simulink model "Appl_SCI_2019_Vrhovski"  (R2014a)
settings: Solver=ode45  StartTime=0.0  StopTime=1000  MaxStep=0.01  RelTol=1e-3
undefined symbols (not defined in the file): deg, H, kg, m, M, mm, N, rad, s, X, Y, Z
libraries: sm_lib x389, nesl_utility x69, simulink x7
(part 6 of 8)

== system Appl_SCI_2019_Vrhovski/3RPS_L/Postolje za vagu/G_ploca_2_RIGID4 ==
  ReferenceFrame : sm_lib/Frames and Transforms/Reference Frame  BlockFunction=simmechanics.library.frames_transforms.reference_frame
  Solid : sm_lib/Body Elements/Solid  InertiaType=Custom  Mass=5  MassUnits=kg  CenterOfMass=[-1.0925911726464245e-05 0 -4.4436244658035022]  CenterOfMassUnits=mm  MomentsOfInertia=[45540 79860 45540]  MomentsOfInertiaUnits=kg*mm^2  ProductsOfInertia=[0 -0.00010369999054466602 0]  ProductsOfInertiaUnits=kg*mm^2  DensityBased=on  Density=1000  DensityUnits=kg/(m^3)  GraphicType=FromGeometry  MarkerShape=Sphere  MarkerSize=10  MarkerSizeUnits=m  GraphicVisPropType=SimpleVisualProperties  GraphicDiffuseColor=[0.8 0.8 0.8]  GraphicSpecularColor=[0.5 0.5 0.5 1.0]  GraphicAmbientColor=[0.15 0.15 0.15 1.0]  GraphicEmissiveColor=[0.0 0.0 0.0 1.0]  GraphicShininess=75  GraphicOpacity=1  GeometryShape=Brick  RectangleSize=[1 1]  RectangleSizeUnits=m  BrickDimensions=[100 65 40]  BrickDimensionUnits=mm  CylinderRadius=120  CylinderRadiusUnits=mm  CylinderLength=20  CylinderLengthUnits=mm  SphereRadius=1  SphereRadiusUnits=m  EllipsoidRadii=[1 1 1]  EllipsoidRadiiUnits=m  ExtrusionCrossSection=[1 1; -1 1; -1 -1; 1 -1]  ExtrusionCrossSectionUnits=m  ExtrusionLength=1  ExtrusionLengthUnits=m  PolygonNumSides=3  PolygonOuterRadius=1  PolygonOuterRadiusUnits=m  ExtGeomFileType=STL  ExtGeomFileName=G_ploca_Default_sldprt.STL  ExtGeomFileUnits=mm  RevolutionCrossSection=[1 1; 1 -1; 2 -1; 2 1]  RevolutionCrossSectionUnits=m  RevolutionExtent=Full  RevolutionAngle=180  RevolutionAngleUnits=deg  BlockFunction=simmechanics.library.body_elements.solid
  Transform1 : sm_lib/Frames and Transforms/Rigid Transform  TranslationMethod=None  TranslationLengthUnit=mm  TranslationStandardAxis=-Z  TranslationStandardOffset=35.5  TranslationCartesianOffset="[-50.0000   86.6025         -10]"  TranslationROffset=0  TranslationROffsetUnits=m  TranslationZOffset=0  TranslationZOffsetUnits=m  TranslationThetaOffset=0  TranslationThetaOffsetUnits=deg  RotationMethod=ArbitraryAxis  RotationAngleUnits=rad  RotationStandardAxis=+Z  RotationAngle=0  RotationArbitraryAxis=[0 0 0]  FollAlignAxisA=+X  BaseAlignAxisA=+Y  FollAlignAxisB=+Y  BaseAlignAxisB=+Z  BlockFunction=simmechanics.library.frames_transforms.rigid_transform
  Transform3 : sm_lib/Frames and Transforms/Rigid Transform  TranslationMethod=None  TranslationLengthUnit=mm  TranslationStandardAxis=+Z  TranslationStandardOffset=35.5  TranslationCartesianOffset=[80.000000000002558 4.2632564145606011e-14 -32.999999999999048]  TranslationROffset=0  TranslationROffsetUnits=m  TranslationZOffset=0  TranslationZOffsetUnits=m  TranslationThetaOffset=0  TranslationThetaOffsetUnits=deg  RotationMethod=None  RotationAngleUnits=rad  RotationStandardAxis=+Z  RotationAngle=0  RotationArbitraryAxis=[0 0 0]  FollAlignAxisA=+X  BaseAlignAxisA=+Y  FollAlignAxisB=+Y  BaseAlignAxisB=+Z  BlockFunction=simmechanics.library.frames_transforms.rigid_transform
  B : PMIOPort  Port=1  Side=Left
  F : PMIOPort  Port=2  Side=Right
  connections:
  Transform3/RConn1 -- F/RConn1
  Transform3/LConn1 -- Solid/RConn1 -- ReferenceFrame/RConn1 -- Transform1/LConn1
  Transform1/RConn1 -- B/RConn1

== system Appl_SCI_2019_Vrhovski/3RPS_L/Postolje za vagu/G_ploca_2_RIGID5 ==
  ReferenceFrame : sm_lib/Frames and Transforms/Reference Frame  BlockFunction=simmechanics.library.frames_transforms.reference_frame
  Solid : sm_lib/Body Elements/Solid  InertiaType=Custom  Mass=5  MassUnits=kg  CenterOfMass=[-1.0925911726464245e-05 0 -4.4436244658035022]  CenterOfMassUnits=mm  MomentsOfInertia=[45540 79860 45540]  MomentsOfInertiaUnits=kg*mm^2  ProductsOfInertia=[0 -0.00010369999054466602 0]  ProductsOfInertiaUnits=kg*mm^2  DensityBased=on  Density=1000  DensityUnits=kg/(m^3)  GraphicType=FromGeometry  MarkerShape=Sphere  MarkerSize=10  MarkerSizeUnits=m  GraphicVisPropType=SimpleVisualProperties  GraphicDiffuseColor=[0.8 0.8 0.8]  GraphicSpecularColor=[0.5 0.5 0.5 1.0]  GraphicAmbientColor=[0.15 0.15 0.15 1.0]  GraphicEmissiveColor=[0.0 0.0 0.0 1.0]  GraphicShininess=75  GraphicOpacity=1  GeometryShape=Brick  RectangleSize=[1 1]  RectangleSizeUnits=m  BrickDimensions=[100 65 40]  BrickDimensionUnits=mm  CylinderRadius=120  CylinderRadiusUnits=mm  CylinderLength=20  CylinderLengthUnits=mm  SphereRadius=1  SphereRadiusUnits=m  EllipsoidRadii=[1 1 1]  EllipsoidRadiiUnits=m  ExtrusionCrossSection=[1 1; -1 1; -1 -1; 1 -1]  ExtrusionCrossSectionUnits=m  ExtrusionLength=1  ExtrusionLengthUnits=m  PolygonNumSides=3  PolygonOuterRadius=1  PolygonOuterRadiusUnits=m  ExtGeomFileType=STL  ExtGeomFileName=G_ploca_Default_sldprt.STL  ExtGeomFileUnits=mm  RevolutionCrossSection=[1 1; 1 -1; 2 -1; 2 1]  RevolutionCrossSectionUnits=m  RevolutionExtent=Full  RevolutionAngle=180  RevolutionAngleUnits=deg  BlockFunction=simmechanics.library.body_elements.solid
  Transform1 : sm_lib/Frames and Transforms/Rigid Transform  TranslationMethod=None  TranslationLengthUnit=mm  TranslationStandardAxis=-Z  TranslationStandardOffset=35.5  TranslationCartesianOffset="[-50.0000   86.6025         -10]"  TranslationROffset=0  TranslationROffsetUnits=m  TranslationZOffset=0  TranslationZOffsetUnits=m  TranslationThetaOffset=0  TranslationThetaOffsetUnits=deg  RotationMethod=ArbitraryAxis  RotationAngleUnits=rad  RotationStandardAxis=+Z  RotationAngle=0  RotationArbitraryAxis=[0 0 0]  FollAlignAxisA=+X  BaseAlignAxisA=+Y  FollAlignAxisB=+Y  BaseAlignAxisB=+Z  BlockFunction=simmechanics.library.frames_transforms.rigid_transform
  Transform3 : sm_lib/Frames and Transforms/Rigid Transform  TranslationMethod=None  TranslationLengthUnit=mm  TranslationStandardAxis=+Z  TranslationStandardOffset=35.5  TranslationCartesianOffset=[80.000000000002558 4.2632564145606011e-14 -32.999999999999048]  TranslationROffset=0  TranslationROffsetUnits=m  TranslationZOffset=0  TranslationZOffsetUnits=m  TranslationThetaOffset=0  TranslationThetaOffsetUnits=deg  RotationMethod=None  RotationAngleUnits=rad  RotationStandardAxis=+Z  RotationAngle=0  RotationArbitraryAxis=[0 0 0]  FollAlignAxisA=+X  BaseAlignAxisA=+Y  FollAlignAxisB=+Y  BaseAlignAxisB=+Z  BlockFunction=simmechanics.library.frames_transforms.rigid_transform
  B : PMIOPort  Port=1  Side=Left
  F : PMIOPort  Port=2  Side=Right
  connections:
  Transform1/RConn1 -- B/RConn1
  Transform1/LConn1 -- ReferenceFrame/RConn1 -- Solid/RConn1 -- Transform3/LConn1
  Transform3/RConn1 -- F/RConn1

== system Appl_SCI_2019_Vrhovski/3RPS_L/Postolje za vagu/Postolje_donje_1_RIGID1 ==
  ReferenceFrame : sm_lib/Frames and Transforms/Reference Frame  BlockFunction=simmechanics.library.frames_transforms.reference_frame
  Transform1 : sm_lib/Frames and Transforms/Rigid Transform  TranslationMethod=Cartesian  TranslationLengthUnit=mm  TranslationStandardAxis=+Z  TranslationStandardOffset=0  TranslationCartesianOffset=[-87.5 72.7 20]  TranslationROffset=0  TranslationROffsetUnits=m  TranslationZOffset=0  TranslationZOffsetUnits=m  TranslationThetaOffset=0  TranslationThetaOffsetUnits=deg  RotationMethod=None  RotationAngleUnits=rad  RotationStandardAxis=+Z  RotationAngle=2.0943951023931975  RotationArbitraryAxis=[0.57735026918962651 -0.57735026918962651 0.5773502691896244]  FollAlignAxisA=+X  BaseAlignAxisA=+Y  FollAlignAxisB=+Y  BaseAlignAxisB=+Z  BlockFunction=simmechanics.library.frames_transforms.rigid_transform
  Transform2 : sm_lib/Frames and Transforms/Rigid Transform  TranslationMethod=Cartesian  TranslationLengthUnit=mm  TranslationStandardAxis=+Z  TranslationStandardOffset=0  TranslationCartesianOffset=[87.5 72.7 20]  TranslationROffset=0  TranslationROffsetUnits=m  TranslationZOffset=0  TranslationZOffsetUnits=m  TranslationThetaOffset=0  TranslationThetaOffsetUnits=deg  RotationMethod=None  RotationAngleUnits=rad  RotationStandardAxis=+Z  RotationAngle=2.0943951023931975  RotationArbitraryAxis=[0.57735026918962651 -0.57735026918962651 0.5773502691896244]  FollAlignAxisA=+X  BaseAlignAxisA=+Y  FollAlignAxisB=+Y  BaseAlignAxisB=+Z  BlockFunction=simmechanics.library.frames_transforms.rigid_transform
  Transform3 : sm_lib/Frames and Transforms/Rigid Transform  TranslationMethod=Cartesian  TranslationLengthUnit=mm  TranslationStandardAxis=+Z  TranslationStandardOffset=0  TranslationCartesianOffset=[-87.5 -72.7 20]  TranslationROffset=0  TranslationROffsetUnits=m  TranslationZOffset=0  TranslationZOffsetUnits=m  TranslationThetaOffset=0  TranslationThetaOffsetUnits=deg  RotationMethod=None  RotationAngleUnits=rad  RotationStandardAxis=+Z  RotationAngle=2.0943951023931975  RotationArbitraryAxis=[0.57735026918962651 -0.57735026918962651 0.5773502691896244]  FollAlignAxisA=+X  BaseAlignAxisA=+Y  FollAlignAxisB=+Y  BaseAlignAxisB=+Z  BlockFunction=simmechanics.library.frames_transforms.rigid_transform
  Transform4 : sm_lib/Frames and Transforms/Rigid Transform  TranslationMethod=Cartesian  TranslationLengthUnit=mm  TranslationStandardAxis=+Z  TranslationStandardOffset=0  TranslationCartesianOffset=[87.5 -72.7 20]  TranslationROffset=0  TranslationROffsetUnits=m  TranslationZOffset=0  TranslationZOffsetUnits=m  TranslationThetaOffset=0  TranslationThetaOffsetUnits=deg  RotationMethod=None  RotationAngleUnits=rad  RotationStandardAxis=+Z  RotationAngle=2.0943951023931975  RotationArbitraryAxis=[0.57735026918962651 -0.57735026918962651 0.5773502691896244]  FollAlignAxisA=+X  BaseAlignAxisA=+Y  FollAlignAxisB=+Y  BaseAlignAxisB=+Z  BlockFunction=simmechanics.library.frames_transforms.rigid_transform
  B : PMIOPort  Port=1  Side=Left
  F1 : PMIOPort  Port=2  Side=Right
  F2 : PMIOPort  Port=3  Side=Right
  F3 : PMIOPort  Port=4  Side=Right
  F4 : PMIOPort  Port=5  Side=Right
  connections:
  ReferenceFrame/RConn1 -- B/RConn1 -- Transform2/LConn1 -- Transform4/LConn1 -- Transform3/LConn1 -- Transform1/LConn1
  F1/RConn1 -- Transform2/RConn1
  Transform1/RConn1 -- F2/RConn1
  Transform3/RConn1 -- F3/RConn1
  Transform4/RConn1 -- F4/RConn1

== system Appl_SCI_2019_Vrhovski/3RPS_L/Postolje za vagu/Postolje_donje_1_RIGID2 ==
  ReferenceFrame : sm_lib/Frames and Transforms/Reference Frame  BlockFunction=simmechanics.library.frames_transforms.reference_frame
  Transform1 : sm_lib/Frames and Transforms/Rigid Transform  TranslationMethod=Cartesian  TranslationLengthUnit=mm  TranslationStandardAxis=+Z  TranslationStandardOffset=10  TranslationCartesianOffset=[-87.5 72.7 0]  TranslationROffset=0  TranslationROffsetUnits=m  TranslationZOffset=0  TranslationZOffsetUnits=m  TranslationThetaOffset=0  TranslationThetaOffsetUnits=deg  RotationMethod=None  RotationAngleUnits=rad  RotationStandardAxis=+Z  RotationAngle=0  RotationArbitraryAxis=[0 0 0]  FollAlignAxisA=+X  BaseAlignAxisA=+Y  FollAlignAxisB=+Y  BaseAlignAxisB=+Z  BlockFunction=simmechanics.library.frames_transforms.rigid_transform
  Transform2 : sm_lib/Frames and Transforms/Rigid Transform  TranslationMethod=Cartesian  TranslationLengthUnit=mm  TranslationStandardAxis=+Z  TranslationStandardOffset=10  TranslationCartesianOffset=[-87.5 -72.7 0]  TranslationROffset=0  TranslationROffsetUnits=m  TranslationZOffset=0  TranslationZOffsetUnits=m  TranslationThetaOffset=0  TranslationThetaOffsetUnits=deg  RotationMethod=None  RotationAngleUnits=rad  RotationStandardAxis=+Z  RotationAngle=0  RotationArbitraryAxis=[0 0 0]  FollAlignAxisA=+X  BaseAlignAxisA=+Y  FollAlignAxisB=+Y  BaseAlignAxisB=+Z  BlockFunction=simmechanics.library.frames_transforms.rigid_transform
  Transform3 : sm_lib/Frames and Transforms/Rigid Transform  TranslationMethod=Cartesian  TranslationLengthUnit=mm  TranslationStandardAxis=+Z  TranslationStandardOffset=10  TranslationCartesianOffset=[87.5 -72.7 0]  TranslationROffset=0  TranslationROffsetUnits=m  TranslationZOffset=0  TranslationZOffsetUnits=m  TranslationThetaOffset=0  TranslationThetaOffsetUnits=deg  RotationMethod=None  RotationAngleUnits=rad  RotationStandardAxis=+Z  RotationAngle=0  RotationArbitraryAxis=[0 0 0]  FollAlignAxisA=+X  BaseAlignAxisA=+Y  FollAlignAxisB=+Y  BaseAlignAxisB=+Z  BlockFunction=simmechanics.library.frames_transforms.rigid_transform
  Transform5 : sm_lib/Frames and Transforms/Rigid Transform  TranslationMethod=Cartesian  TranslationLengthUnit=mm  TranslationStandardAxis=+Z  TranslationStandardOffset=10  TranslationCartesianOffset=[87.5 72.7 0]  TranslationROffset=0  TranslationROffsetUnits=m  TranslationZOffset=0  TranslationZOffsetUnits=m  TranslationThetaOffset=0  TranslationThetaOffsetUnits=deg  RotationMethod=None  RotationAngleUnits=rad  RotationStandardAxis=+Z  RotationAngle=0  RotationArbitraryAxis=[0 0 0]  FollAlignAxisA=+X  BaseAlignAxisA=+Y  FollAlignAxisB=+Y  BaseAlignAxisB=+Z  BlockFunction=simmechanics.library.frames_transforms.rigid_transform
  B : PMIOPort  Port=1  Side=Right
  F1 : PMIOPort  Port=2  Side=Left
  F2 : PMIOPort  Port=3  Side=Left
  F3 : PMIOPort  Port=4  Side=Left
  F4 : PMIOPort  Port=5  Side=Left
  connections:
  ReferenceFrame/RConn1 -- Transform1/LConn1 -- Transform3/LConn1 -- Transform2/LConn1 -- B/RConn1 -- Transform5/LConn1
  Transform1/RConn1 -- F2/RConn1
  Transform2/RConn1 -- F3/RConn1
  Transform3/RConn1 -- F4/RConn1
  Transform5/RConn1 -- F1/RConn1

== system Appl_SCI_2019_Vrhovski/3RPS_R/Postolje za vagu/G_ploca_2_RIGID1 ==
  ReferenceFrame : sm_lib/Frames and Transforms/Reference Frame  BlockFunction=simmechanics.library.frames_transforms.reference_frame
  Solid : sm_lib/Body Elements/Solid  InertiaType=Custom  Mass=5  MassUnits=kg  CenterOfMass=[-1.0925911726464245e-05 0 -4.4436244658035022]  CenterOfMassUnits=mm  MomentsOfInertia=[45540 79860 45540]  MomentsOfInertiaUnits=kg*mm^2  ProductsOfInertia=[0 -0.00010369999054466602 0]  ProductsOfInertiaUnits=kg*mm^2  DensityBased=on  Density=1000  DensityUnits=kg/(m^3)  GraphicType=FromGeometry  MarkerShape=Sphere  MarkerSize=10  MarkerSizeUnits=m  GraphicVisPropType=SimpleVisualProperties  GraphicDiffuseColor=[0.8 0.8 0.8]  GraphicSpecularColor=[0.5 0.5 0.5 1.0]  GraphicAmbientColor=[0.15 0.15 0.15 1.0]  GraphicEmissiveColor=[0.0 0.0 0.0 1.0]  GraphicShininess=75  GraphicOpacity=1  GeometryShape=Brick  RectangleSize=[1 1]  RectangleSizeUnits=m  BrickDimensions=[100 65 40]  BrickDimensionUnits=mm  CylinderRadius=120  CylinderRadiusUnits=mm  CylinderLength=20  CylinderLengthUnits=mm  SphereRadius=1  SphereRadiusUnits=m  EllipsoidRadii=[1 1 1]  EllipsoidRadiiUnits=m  ExtrusionCrossSection=[1 1; -1 1; -1 -1; 1 -1]  ExtrusionCrossSectionUnits=m  ExtrusionLength=1  ExtrusionLengthUnits=m  PolygonNumSides=3  PolygonOuterRadius=1  PolygonOuterRadiusUnits=m  ExtGeomFileType=STL  ExtGeomFileName=G_ploca_Default_sldprt.STL  ExtGeomFileUnits=mm  RevolutionCrossSection=[1 1; 1 -1; 2 -1; 2 1]  RevolutionCrossSectionUnits=m  RevolutionExtent=Full  RevolutionAngle=180  RevolutionAngleUnits=deg  BlockFunction=simmechanics.library.body_elements.solid
  Transform1 : sm_lib/Frames and Transforms/Rigid Transform  TranslationMethod=None  TranslationLengthUnit=mm  TranslationStandardAxis=-Z  TranslationStandardOffset=35.5  TranslationCartesianOffset="[-50.0000   86.6025         -10]"  TranslationROffset=0  TranslationROffsetUnits=m  TranslationZOffset=0  TranslationZOffsetUnits=m  TranslationThetaOffset=0  TranslationThetaOffsetUnits=deg  RotationMethod=ArbitraryAxis  RotationAngleUnits=rad  RotationStandardAxis=+Z  RotationAngle=0  RotationArbitraryAxis=[0 0 0]  FollAlignAxisA=+X  BaseAlignAxisA=+Y  FollAlignAxisB=+Y  BaseAlignAxisB=+Z  BlockFunction=simmechanics.library.frames_transforms.rigid_transform
  Transform3 : sm_lib/Frames and Transforms/Rigid Transform  TranslationMethod=None  TranslationLengthUnit=mm  TranslationStandardAxis=+Z  TranslationStandardOffset=35.5  TranslationCartesianOffset=[80.000000000002558 4.2632564145606011e-14 -32.999999999999048]  TranslationROffset=0  TranslationROffsetUnits=m  TranslationZOffset=0  TranslationZOffsetUnits=m  TranslationThetaOffset=0  TranslationThetaOffsetUnits=deg  RotationMethod=None  RotationAngleUnits=rad  RotationStandardAxis=+Z  RotationAngle=0  RotationArbitraryAxis=[0 0 0]  FollAlignAxisA=+X  BaseAlignAxisA=+Y  FollAlignAxisB=+Y  BaseAlignAxisB=+Z  BlockFunction=simmechanics.library.frames_transforms.rigid_transform
  B : PMIOPort  Port=1  Side=Left
  F : PMIOPort  Port=2  Side=Right
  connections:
  Transform3/RConn1 -- F/RConn1
  Solid/RConn1 -- Transform1/LConn1 -- ReferenceFrame/RConn1 -- Transform3/LConn1
  Transform1/RConn1 -- B/RConn1

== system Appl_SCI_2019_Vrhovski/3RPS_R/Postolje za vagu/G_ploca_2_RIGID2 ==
  ReferenceFrame : sm_lib/Frames and Transforms/Reference Frame  BlockFunction=simmechanics.library.frames_transforms.reference_frame
  Solid : sm_lib/Body Elements/Solid  InertiaType=Custom  Mass=5  MassUnits=kg  CenterOfMass=[-1.0925911726464245e-05 0 -4.4436244658035022]  CenterOfMassUnits=mm  MomentsOfInertia=[45540 79860 45540]  MomentsOfInertiaUnits=kg*mm^2  ProductsOfInertia=[0 -0.00010369999054466602 0]  ProductsOfInertiaUnits=kg*mm^2  DensityBased=on  Density=1000  DensityUnits=kg/(m^3)  GraphicType=FromGeometry  MarkerShape=Sphere  MarkerSize=10  MarkerSizeUnits=m  GraphicVisPropType=SimpleVisualProperties  GraphicDiffuseColor=[0.8 0.8 0.8]  GraphicSpecularColor=[0.5 0.5 0.5 1.0]  GraphicAmbientColor=[0.15 0.15 0.15 1.0]  GraphicEmissiveColor=[0.0 0.0 0.0 1.0]  GraphicShininess=75  GraphicOpacity=1  GeometryShape=Brick  RectangleSize=[1 1]  RectangleSizeUnits=m  BrickDimensions=[100 65 40]  BrickDimensionUnits=mm  CylinderRadius=120  CylinderRadiusUnits=mm  CylinderLength=20  CylinderLengthUnits=mm  SphereRadius=1  SphereRadiusUnits=m  EllipsoidRadii=[1 1 1]  EllipsoidRadiiUnits=m  ExtrusionCrossSection=[1 1; -1 1; -1 -1; 1 -1]  ExtrusionCrossSectionUnits=m  ExtrusionLength=1  ExtrusionLengthUnits=m  PolygonNumSides=3  PolygonOuterRadius=1  PolygonOuterRadiusUnits=m  ExtGeomFileType=STL  ExtGeomFileName=G_ploca_Default_sldprt.STL  ExtGeomFileUnits=mm  RevolutionCrossSection=[1 1; 1 -1; 2 -1; 2 1]  RevolutionCrossSectionUnits=m  RevolutionExtent=Full  RevolutionAngle=180  RevolutionAngleUnits=deg  BlockFunction=simmechanics.library.body_elements.solid
  Transform1 : sm_lib/Frames and Transforms/Rigid Transform  TranslationMethod=None  TranslationLengthUnit=mm  TranslationStandardAxis=-Z  TranslationStandardOffset=35.5  TranslationCartesianOffset="[-50.0000   86.6025         -10]"  TranslationROffset=0  TranslationROffsetUnits=m  TranslationZOffset=0  TranslationZOffsetUnits=m  TranslationThetaOffset=0  TranslationThetaOffsetUnits=deg  RotationMethod=ArbitraryAxis  RotationAngleUnits=rad  RotationStandardAxis=+Z  RotationAngle=0  RotationArbitraryAxis=[0 0 0]  FollAlignAxisA=+X  BaseAlignAxisA=+Y  FollAlignAxisB=+Y  BaseAlignAxisB=+Z  BlockFunction=simmechanics.library.frames_transforms.rigid_transform
  Transform3 : sm_lib/Frames and Transforms/Rigid Transform  TranslationMethod=None  TranslationLengthUnit=mm  TranslationStandardAxis=+Z  TranslationStandardOffset=35.5  TranslationCartesianOffset=[80.000000000002558 4.2632564145606011e-14 -32.999999999999048]  TranslationROffset=0  TranslationROffsetUnits=m  TranslationZOffset=0  TranslationZOffsetUnits=m  TranslationThetaOffset=0  TranslationThetaOffsetUnits=deg  RotationMethod=None  RotationAngleUnits=rad  RotationStandardAxis=+Z  RotationAngle=0  RotationArbitraryAxis=[0 0 0]  FollAlignAxisA=+X  BaseAlignAxisA=+Y  FollAlignAxisB=+Y  BaseAlignAxisB=+Z  BlockFunction=simmechanics.library.frames_transforms.rigid_transform
  B : PMIOPort  Port=1  Side=Left
  F : PMIOPort  Port=2  Side=Right
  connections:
  Transform1/RConn1 -- B/RConn1
  Transform1/LConn1 -- ReferenceFrame/RConn1 -- Solid/RConn1 -- Transform3/LConn1
  Transform3/RConn1 -- F/RConn1

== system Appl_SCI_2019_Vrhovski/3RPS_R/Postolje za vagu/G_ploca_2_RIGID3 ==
  ReferenceFrame : sm_lib/Frames and Transforms/Reference Frame  BlockFunction=simmechanics.library.frames_transforms.reference_frame
  Solid : sm_lib/Body Elements/Solid  InertiaType=Custom  Mass=5  MassUnits=kg  CenterOfMass=[-1.0925911726464245e-05 0 -4.4436244658035022]  CenterOfMassUnits=mm  MomentsOfInertia=[45540 79860 45540]  MomentsOfInertiaUnits=kg*mm^2  ProductsOfInertia=[0 -0.00010369999054466602 0]  ProductsOfInertiaUnits=kg*mm^2  DensityBased=on  Density=1000  DensityUnits=kg/(m^3)  GraphicType=FromGeometry  MarkerShape=Sphere  MarkerSize=10  MarkerSizeUnits=m  GraphicVisPropType=SimpleVisualProperties  GraphicDiffuseColor=[0.4 0.4 0.4]  GraphicSpecularColor=[0.5 0.5 0.5 1.0]  GraphicAmbientColor=[0.15 0.15 0.15 1.0]  GraphicEmissiveColor=[0.0 0.0 0.0 1.0]  GraphicShininess=75  GraphicOpacity=1  GeometryShape=Brick  RectangleSize=[1 1]  RectangleSizeUnits=m  BrickDimensions=[380 210 11]  BrickDimensionUnits=mm  CylinderRadius=120  CylinderRadiusUnits=mm  CylinderLength=20  CylinderLengthUnits=mm  SphereRadius=1  SphereRadiusUnits=m  EllipsoidRadii=[1 1 1]  EllipsoidRadiiUnits=m  ExtrusionCrossSection=[1 1; -1 1; -1 -1; 1 -1]  ExtrusionCrossSectionUnits=m  ExtrusionLength=1  ExtrusionLengthUnits=m  PolygonNumSides=3  PolygonOuterRadius=1  PolygonOuterRadiusUnits=m  ExtGeomFileType=STL  ExtGeomFileName=G_ploca_Default_sldprt.STL  ExtGeomFileUnits=mm  RevolutionCrossSection=[1 1; 1 -1; 2 -1; 2 1]  RevolutionCrossSectionUnits=m  RevolutionExtent=Full  RevolutionAngle=180  RevolutionAngleUnits=deg  BlockFunction=simmechanics.library.body_elements.solid
  Transform1 : sm_lib/Frames and Transforms/Rigid Transform  TranslationMethod=StandardAxis  TranslationLengthUnit=mm  TranslationStandardAxis=-Z  TranslationStandardOffset=25.5  TranslationCartesianOffset="[-50.0000   86.6025         -10]"  TranslationROffset=0  TranslationROffsetUnits=m  TranslationZOffset=0  TranslationZOffsetUnits=m  TranslationThetaOffset=0  TranslationThetaOffsetUnits=deg  RotationMethod=ArbitraryAxis  RotationAngleUnits=rad  RotationStandardAxis=+Z  RotationAngle=0  RotationArbitraryAxis=[0 0 0]  FollAlignAxisA=+X  BaseAlignAxisA=+Y  FollAlignAxisB=+Y  BaseAlignAxisB=+Z  BlockFunction=simmechanics.library.frames_transforms.rigid_transform
  Transform3 : sm_lib/Frames and Transforms/Rigid Transform  TranslationMethod=StandardAxis  TranslationLengthUnit=mm  TranslationStandardAxis=+Z  TranslationStandardOffset=5.5  TranslationCartesianOffset=[80.000000000002558 4.2632564145606011e-14 -32.999999999999048]  TranslationROffset=0  TranslationROffsetUnits=m  TranslationZOffset=0  TranslationZOffsetUnits=m  TranslationThetaOffset=0  TranslationThetaOffsetUnits=deg  RotationMethod=None  RotationAngleUnits=rad  RotationStandardAxis=+Z  RotationAngle=0  RotationArbitraryAxis=[0 0 0]  FollAlignAxisA=+X  BaseAlignAxisA=+Y  FollAlignAxisB=+Y  BaseAlignAxisB=+Z  BlockFunction=simmechanics.library.frames_transforms.rigid_transform
  B : PMIOPort  Port=1  Side=Left
  F : PMIOPort  Port=2  Side=Right
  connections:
  Transform3/RConn1 -- F/RConn1
  Transform1/RConn1 -- B/RConn1
  Solid/RConn1 -- Transform3/LConn1 -- Transform1/LConn1 -- ReferenceFrame/RConn1

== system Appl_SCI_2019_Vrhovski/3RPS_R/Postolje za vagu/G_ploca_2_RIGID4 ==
  ReferenceFrame : sm_lib/Frames and Transforms/Reference Frame  BlockFunction=simmechanics.library.frames_transforms.reference_frame
  Solid : sm_lib/Body Elements/Solid  InertiaType=Custom  Mass=5  MassUnits=kg  CenterOfMass=[-1.0925911726464245e-05 0 -4.4436244658035022]  CenterOfMassUnits=mm  MomentsOfInertia=[45540 79860 45540]  MomentsOfInertiaUnits=kg*mm^2  ProductsOfInertia=[0 -0.00010369999054466602 0]  ProductsOfInertiaUnits=kg*mm^2  DensityBased=on  Density=1000  DensityUnits=kg/(m^3)  GraphicType=FromGeometry  MarkerShape=Sphere  MarkerSize=10  MarkerSizeUnits=m  GraphicVisPropType=SimpleVisualProperties  GraphicDiffuseColor=[0.8 0.8 0.8]  GraphicSpecularColor=[0.5 0.5 0.5 1.0]  GraphicAmbientColor=[0.15 0.15 0.15 1.0]  GraphicEmissiveColor=[0.0 0.0 0.0 1.0]  GraphicShininess=75  GraphicOpacity=1  GeometryShape=Brick  RectangleSize=[1 1]  RectangleSizeUnits=m  BrickDimensions=[100 65 40]  BrickDimensionUnits=mm  CylinderRadius=120  CylinderRadiusUnits=mm  CylinderLength=20  CylinderLengthUnits=mm  SphereRadius=1  SphereRadiusUnits=m  EllipsoidRadii=[1 1 1]  EllipsoidRadiiUnits=m  ExtrusionCrossSection=[1 1; -1 1; -1 -1; 1 -1]  ExtrusionCrossSectionUnits=m  ExtrusionLength=1  ExtrusionLengthUnits=m  PolygonNumSides=3  PolygonOuterRadius=1  PolygonOuterRadiusUnits=m  ExtGeomFileType=STL  ExtGeomFileName=G_ploca_Default_sldprt.STL  ExtGeomFileUnits=mm  RevolutionCrossSection=[1 1; 1 -1; 2 -1; 2 1]  RevolutionCrossSectionUnits=m  RevolutionExtent=Full  RevolutionAngle=180  RevolutionAngleUnits=deg  BlockFunction=simmechanics.library.body_elements.solid
  Transform1 : sm_lib/Frames and Transforms/Rigid Transform  TranslationMethod=None  TranslationLengthUnit=mm  TranslationStandardAxis=-Z  TranslationStandardOffset=35.5  TranslationCartesianOffset="[-50.0000   86.6025         -10]"  TranslationROffset=0  TranslationROffsetUnits=m  TranslationZOffset=0  TranslationZOffsetUnits=m  TranslationThetaOffset=0  TranslationThetaOffsetUnits=deg  RotationMethod=ArbitraryAxis  RotationAngleUnits=rad  RotationStandardAxis=+Z  RotationAngle=0  RotationArbitraryAxis=[0 0 0]  FollAlignAxisA=+X  BaseAlignAxisA=+Y  FollAlignAxisB=+Y  BaseAlignAxisB=+Z  BlockFunction=simmechanics.library.frames_transforms.rigid_transform
  Transform3 : sm_lib/Frames and Transforms/Rigid Transform  TranslationMethod=None  TranslationLengthUnit=mm  TranslationStandardAxis=+Z  TranslationStandardOffset=35.5  TranslationCartesianOffset=[80.000000000002558 4.2632564145606011e-14 -32.999999999999048]  TranslationROffset=0  TranslationROffsetUnits=m  TranslationZOffset=0  TranslationZOffsetUnits=m  TranslationThetaOffset=0  TranslationThetaOffsetUnits=deg  RotationMethod=None  RotationAngleUnits=rad  RotationStandardAxis=+Z  RotationAngle=0  RotationArbitraryAxis=[0 0 0]  FollAlignAxisA=+X  BaseAlignAxisA=+Y  FollAlignAxisB=+Y  BaseAlignAxisB=+Z  BlockFunction=simmechanics.library.frames_transforms.rigid_transform
  B : PMIOPort  Port=1  Side=Left
  F : PMIOPort  Port=2  Side=Right
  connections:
  Transform3/RConn1 -- F/RConn1
  Transform3/LConn1 -- Solid/RConn1 -- ReferenceFrame/RConn1 -- Transform1/LConn1
  Transform1/RConn1 -- B/RConn1

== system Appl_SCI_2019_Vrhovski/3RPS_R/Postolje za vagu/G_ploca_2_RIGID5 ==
  ReferenceFrame : sm_lib/Frames and Transforms/Reference Frame  BlockFunction=simmechanics.library.frames_transforms.reference_frame
  Solid : sm_lib/Body Elements/Solid  InertiaType=Custom  Mass=5  MassUnits=kg  CenterOfMass=[-1.0925911726464245e-05 0 -4.4436244658035022]  CenterOfMassUnits=mm  MomentsOfInertia=[45540 79860 45540]  MomentsOfInertiaUnits=kg*mm^2  ProductsOfInertia=[0 -0.00010369999054466602 0]  ProductsOfInertiaUnits=kg*mm^2  DensityBased=on  Density=1000  DensityUnits=kg/(m^3)  GraphicType=FromGeometry  MarkerShape=Sphere  MarkerSize=10  MarkerSizeUnits=m  GraphicVisPropType=SimpleVisualProperties  GraphicDiffuseColor=[0.8 0.8 0.8]  GraphicSpecularColor=[0.5 0.5 0.5 1.0]  GraphicAmbientColor=[0.15 0.15 0.15 1.0]  GraphicEmissiveColor=[0.0 0.0 0.0 1.0]  GraphicShininess=75  GraphicOpacity=1  GeometryShape=Brick  RectangleSize=[1 1]  RectangleSizeUnits=m  BrickDimensions=[100 65 40]  BrickDimensionUnits=mm  CylinderRadius=120  CylinderRadiusUnits=mm  CylinderLength=20  CylinderLengthUnits=mm  SphereRadius=1  SphereRadiusUnits=m  EllipsoidRadii=[1 1 1]  EllipsoidRadiiUnits=m  ExtrusionCrossSection=[1 1; -1 1; -1 -1; 1 -1]  ExtrusionCrossSectionUnits=m  ExtrusionLength=1  ExtrusionLengthUnits=m  PolygonNumSides=3  PolygonOuterRadius=1  PolygonOuterRadiusUnits=m  ExtGeomFileType=STL  ExtGeomFileName=G_ploca_Default_sldprt.STL  ExtGeomFileUnits=mm  RevolutionCrossSection=[1 1; 1 -1; 2 -1; 2 1]  RevolutionCrossSectionUnits=m  RevolutionExtent=Full  RevolutionAngle=180  RevolutionAngleUnits=deg  BlockFunction=simmechanics.library.body_elements.solid
  Transform1 : sm_lib/Frames and Transforms/Rigid Transform  TranslationMethod=None  TranslationLengthUnit=mm  TranslationStandardAxis=-Z  TranslationStandardOffset=35.5  TranslationCartesianOffset="[-50.0000   86.6025         -10]"  TranslationROffset=0  TranslationROffsetUnits=m  TranslationZOffset=0  TranslationZOffsetUnits=m  TranslationThetaOffset=0  TranslationThetaOffsetUnits=deg  RotationMethod=ArbitraryAxis  RotationAngleUnits=rad  RotationStandardAxis=+Z  RotationAngle=0  RotationArbitraryAxis=[0 0 0]  FollAlignAxisA=+X  BaseAlignAxisA=+Y  FollAlignAxisB=+Y  BaseAlignAxisB=+Z  BlockFunction=simmechanics.library.frames_transforms.rigid_transform
  Transform3 : sm_lib/Frames and Transforms/Rigid Transform  TranslationMethod=None  TranslationLengthUnit=mm  TranslationStandardAxis=+Z  TranslationStandardOffset=35.5  TranslationCartesianOffset=[80.000000000002558 4.2632564145606011e-14 -32.999999999999048]  TranslationROffset=0  TranslationROffsetUnits=m  TranslationZOffset=0  TranslationZOffsetUnits=m  TranslationThetaOffset=0  TranslationThetaOffsetUnits=deg  RotationMethod=None  RotationAngleUnits=rad  RotationStandardAxis=+Z  RotationAngle=0  RotationArbitraryAxis=[0 0 0]  FollAlignAxisA=+X  BaseAlignAxisA=+Y  FollAlignAxisB=+Y  BaseAlignAxisB=+Z  BlockFunction=simmechanics.library.frames_transforms.rigid_transform
  B : PMIOPort  Port=1  Side=Left
  F : PMIOPort  Port=2  Side=Right
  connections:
  Transform1/RConn1 -- B/RConn1
  Transform1/LConn1 -- ReferenceFrame/RConn1 -- Solid/RConn1 -- Transform3/LConn1
  Transform3/RConn1 -- F/RConn1

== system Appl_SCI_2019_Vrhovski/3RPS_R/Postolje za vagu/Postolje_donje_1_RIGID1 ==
  ReferenceFrame : sm_lib/Frames and Transforms/Reference Frame  BlockFunction=simmechanics.library.frames_transforms.reference_frame
  Transform1 : sm_lib/Frames and Transforms/Rigid Transform  TranslationMethod=Cartesian  TranslationLengthUnit=mm  TranslationStandardAxis=+Z  TranslationStandardOffset=0  TranslationCartesianOffset=[-87.5 72.7 20]  TranslationROffset=0  TranslationROffsetUnits=m  TranslationZOffset=0  TranslationZOffsetUnits=m  TranslationThetaOffset=0  TranslationThetaOffsetUnits=deg  RotationMethod=None  RotationAngleUnits=rad  RotationStandardAxis=+Z  RotationAngle=2.0943951023931975  RotationArbitraryAxis=[0.57735026918962651 -0.57735026918962651 0.5773502691896244]  FollAlignAxisA=+X  BaseAlignAxisA=+Y  FollAlignAxisB=+Y  BaseAlignAxisB=+Z  BlockFunction=simmechanics.library.frames_transforms.rigid_transform
  Transform2 : sm_lib/Frames and Transforms/Rigid Transform  TranslationMethod=Cartesian  TranslationLengthUnit=mm  TranslationStandardAxis=+Z  TranslationStandardOffset=0  TranslationCartesianOffset=[87.5 72.7 20]  TranslationROffset=0  TranslationROffsetUnits=m  TranslationZOffset=0  TranslationZOffsetUnits=m  TranslationThetaOffset=0  TranslationThetaOffsetUnits=deg  RotationMethod=None  RotationAngleUnits=rad  RotationStandardAxis=+Z  RotationAngle=2.0943951023931975  RotationArbitraryAxis=[0.57735026918962651 -0.57735026918962651 0.5773502691896244]  FollAlignAxisA=+X  BaseAlignAxisA=+Y  FollAlignAxisB=+Y  BaseAlignAxisB=+Z  BlockFunction=simmechanics.library.frames_transforms.rigid_transform
  Transform3 : sm_lib/Frames and Transforms/Rigid Transform  TranslationMethod=Cartesian  TranslationLengthUnit=mm  TranslationStandardAxis=+Z  TranslationStandardOffset=0  TranslationCartesianOffset=[-87.5 -72.7 20]  TranslationROffset=0  TranslationROffsetUnits=m  TranslationZOffset=0  TranslationZOffsetUnits=m  TranslationThetaOffset=0  TranslationThetaOffsetUnits=deg  RotationMethod=None  RotationAngleUnits=rad  RotationStandardAxis=+Z  RotationAngle=2.0943951023931975  RotationArbitraryAxis=[0.57735026918962651 -0.57735026918962651 0.5773502691896244]  FollAlignAxisA=+X  BaseAlignAxisA=+Y  FollAlignAxisB=+Y  BaseAlignAxisB=+Z  BlockFunction=simmechanics.library.frames_transforms.rigid_transform
  Transform4 : sm_lib/Frames and Transforms/Rigid Transform  TranslationMethod=Cartesian  TranslationLengthUnit=mm  TranslationStandardAxis=+Z  TranslationStandardOffset=0  TranslationCartesianOffset=[87.5 -72.7 20]  TranslationROffset=0  TranslationROffsetUnits=m  TranslationZOffset=0  TranslationZOffsetUnits=m  TranslationThetaOffset=0  TranslationThetaOffsetUnits=deg  RotationMethod=None  RotationAngleUnits=rad  RotationStandardAxis=+Z  RotationAngle=2.0943951023931975  RotationArbitraryAxis=[0.57735026918962651 -0.57735026918962651 0.5773502691896244]  FollAlignAxisA=+X  BaseAlignAxisA=+Y  FollAlignAxisB=+Y  BaseAlignAxisB=+Z  BlockFunction=simmechanics.library.frames_transforms.rigid_transform
  B : PMIOPort  Port=1  Side=Left
  F1 : PMIOPort  Port=2  Side=Right
  F2 : PMIOPort  Port=3  Side=Right
  F3 : PMIOPort  Port=4  Side=Right
  F4 : PMIOPort  Port=5  Side=Right
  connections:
  ReferenceFrame/RConn1 -- B/RConn1 -- Transform2/LConn1 -- Transform4/LConn1 -- Transform3/LConn1 -- Transform1/LConn1
  F1/RConn1 -- Transform2/RConn1
  Transform1/RConn1 -- F2/RConn1
  Transform3/RConn1 -- F3/RConn1
  Transform4/RConn1 -- F4/RConn1

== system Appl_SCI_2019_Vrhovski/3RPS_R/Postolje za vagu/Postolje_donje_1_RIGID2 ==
  ReferenceFrame : sm_lib/Frames and Transforms/Reference Frame  BlockFunction=simmechanics.library.frames_transforms.reference_frame
  Transform1 : sm_lib/Frames and Transforms/Rigid Transform  TranslationMethod=Cartesian  TranslationLengthUnit=mm  TranslationStandardAxis=+Z  TranslationStandardOffset=10  TranslationCartesianOffset=[-87.5 72.7 0]  TranslationROffset=0  TranslationROffsetUnits=m  TranslationZOffset=0  TranslationZOffsetUnits=m  TranslationThetaOffset=0  TranslationThetaOffsetUnits=deg  RotationMethod=None  RotationAngleUnits=rad  RotationStandardAxis=+Z  RotationAngle=0  RotationArbitraryAxis=[0 0 0]  FollAlignAxisA=+X  BaseAlignAxisA=+Y  FollAlignAxisB=+Y  BaseAlignAxisB=+Z  BlockFunction=simmechanics.library.frames_transforms.rigid_transform
  Transform2 : sm_lib/Frames and Transforms/Rigid Transform  TranslationMethod=Cartesian  TranslationLengthUnit=mm  TranslationStandardAxis=+Z  TranslationStandardOffset=10  TranslationCartesianOffset=[-87.5 -72.7 0]  TranslationROffset=0  TranslationROffsetUnits=m  TranslationZOffset=0  TranslationZOffsetUnits=m  TranslationThetaOffset=0  TranslationThetaOffsetUnits=deg  RotationMethod=None  RotationAngleUnits=rad  RotationStandardAxis=+Z  RotationAngle=0  RotationArbitraryAxis=[0 0 0]  FollAlignAxisA=+X  BaseAlignAxisA=+Y  FollAlignAxisB=+Y  BaseAlignAxisB=+Z  BlockFunction=simmechanics.library.frames_transforms.rigid_transform
  Transform3 : sm_lib/Frames and Transforms/Rigid Transform  TranslationMethod=Cartesian  TranslationLengthUnit=mm  TranslationStandardAxis=+Z  TranslationStandardOffset=10  TranslationCartesianOffset=[87.5 -72.7 0]  TranslationROffset=0  TranslationROffsetUnits=m  TranslationZOffset=0  TranslationZOffsetUnits=m  TranslationThetaOffset=0  TranslationThetaOffsetUnits=deg  RotationMethod=None  RotationAngleUnits=rad  RotationStandardAxis=+Z  RotationAngle=0  RotationArbitraryAxis=[0 0 0]  FollAlignAxisA=+X  BaseAlignAxisA=+Y  FollAlignAxisB=+Y  BaseAlignAxisB=+Z  BlockFunction=simmechanics.library.frames_transforms.rigid_transform
  Transform5 : sm_lib/Frames and Transforms/Rigid Transform  TranslationMethod=Cartesian  TranslationLengthUnit=mm  TranslationStandardAxis=+Z  TranslationStandardOffset=10  TranslationCartesianOffset=[87.5 72.7 0]  TranslationROffset=0  TranslationROffsetUnits=m  TranslationZOffset=0  TranslationZOffsetUnits=m  TranslationThetaOffset=0  TranslationThetaOffsetUnits=deg  RotationMethod=None  RotationAngleUnits=rad  RotationStandardAxis=+Z  RotationAngle=0  RotationArbitraryAxis=[0 0 0]  FollAlignAxisA=+X  BaseAlignAxisA=+Y  FollAlignAxisB=+Y  BaseAlignAxisB=+Z  BlockFunction=simmechanics.library.frames_transforms.rigid_transform
  B : PMIOPort  Port=1  Side=Right
  F1 : PMIOPort  Port=2  Side=Left
  F2 : PMIOPort  Port=3  Side=Left
  F3 : PMIOPort  Port=4  Side=Left
  F4 : PMIOPort  Port=5  Side=Left
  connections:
  ReferenceFrame/RConn1 -- Transform1/LConn1 -- Transform3/LConn1 -- Transform2/LConn1 -- B/RConn1 -- Transform5/LConn1
  Transform1/RConn1 -- F2/RConn1
  Transform2/RConn1 -- F3/RConn1
  Transform3/RConn1 -- F4/RConn1
  Transform5/RConn1 -- F1/RConn1

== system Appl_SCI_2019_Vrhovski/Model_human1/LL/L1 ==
  Mux : Mux  Inputs=3
  Pos X Converter : nesl_utility/PS-Simulink Converter  PhysicalDomain=network_engine_domain  SubClassName=ps_output  LeftPortType=input  RightPortType=output  PseudoPeriodic=off  Frequencies=[]  Unit=mm  AffineConversion=off
  Pos Y Converter : nesl_utility/PS-Simulink Converter  PhysicalDomain=network_engine_domain  SubClassName=ps_output  LeftPortType=input  RightPortType=output  PseudoPeriodic=off  Frequencies=[]  Unit=mm  AffineConversion=off
  Pos Z Converter2 : nesl_utility/PS-Simulink Converter  PhysicalDomain=network_engine_domain  SubClassName=ps_output  LeftPortType=input  RightPortType=output  PseudoPeriodic=off  Frequencies=[]  Unit=mm  AffineConversion=off
  Transform Sensor : sm_lib/Frames and Transforms/Transform Sensor  MeasurementFrame=World  SenseAngle=off  SenseAxis=off  SenseAngle1=off  SenseAngle2=off  SenseAngle3=off  SenseQ=off  SenseR=off  SenseOmegaX=off  SenseOmegaY=off  SenseOmegaZ=off  SenseOmega1=off  SenseOmega2=off  SenseOmega3=off  SenseQDot=off  SenseRDot=off  SenseAlphaX=off  SenseAlphaY=off  SenseAlphaZ=off  SenseAlpha1=off  SenseAlpha2=off  SenseAlpha3=off  SenseQDDot=off  SenseRDDot=off  SenseX=on  SenseY=on  SenseZ=on  SenseRad=on  SenseAzim=off  SenseDist=off  SenseInc=off  SenseXDot=off  SenseYDot=off  SenseZDot=off  SenseRadDot=off  SenseAzimDot=off  SenseDistDot=off  SenseIncDot=off  SenseXDDot=off  SenseYDDot=off  SenseZDDot=off  SenseRadDDot=off  SenseAzimDDot=off  SenseDistDDot=off  SenseIncDDot=off  BlockFunction=simmechanics.library.frames_transforms.transform_sensor
  base_coord_sys : PMIOPort  Port=1  Side=Left
  marker : PMIOPort  Port=2  Side=Left
  xyz : Outport
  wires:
  Pos Z Converter2/1 -> Mux/3
  Pos X Converter/1 -> Mux/1
  Pos Y Converter/1 -> Mux/2
  Mux/1 -> xyz/1
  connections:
  base_coord_sys/RConn1 -- Transform Sensor/LConn1
  marker/RConn1 -- Transform Sensor/RConn1
  Pos Z Converter2/LConn1 -- Transform Sensor/RConn4
  Pos X Converter/LConn1 -- Transform Sensor/RConn2
  Transform Sensor/RConn3 -- Pos Y Converter/LConn1

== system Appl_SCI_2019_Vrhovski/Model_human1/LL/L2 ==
  Mux : Mux  Inputs=3
  Pos X Converter : nesl_utility/PS-Simulink Converter  PhysicalDomain=network_engine_domain  SubClassName=ps_output  LeftPortType=input  RightPortType=output  PseudoPeriodic=off  Frequencies=[]  Unit=mm  AffineConversion=off
  Pos Y Converter : nesl_utility/PS-Simulink Converter  PhysicalDomain=network_engine_domain  SubClassName=ps_output  LeftPortType=input  RightPortType=output  PseudoPeriodic=off  Frequencies=[]  Unit=mm  AffineConversion=off
  Pos Z Converter2 : nesl_utility/PS-Simulink Converter  PhysicalDomain=network_engine_domain  SubClassName=ps_output  LeftPortType=input  RightPortType=output  PseudoPeriodic=off  Frequencies=[]  Unit=mm  AffineConversion=off
  Transform Sensor : sm_lib/Frames and Transforms/Transform Sensor  MeasurementFrame=World  SenseAngle=off  SenseAxis=off  SenseAngle1=off  SenseAngle2=off  SenseAngle3=off  SenseQ=off  SenseR=off  SenseOmegaX=off  SenseOmegaY=off  SenseOmegaZ=off  SenseOmega1=off  SenseOmega2=off  SenseOmega3=off  SenseQDot=off  SenseRDot=off  SenseAlphaX=off  SenseAlphaY=off  SenseAlphaZ=off  SenseAlpha1=off  SenseAlpha2=off  SenseAlpha3=off  SenseQDDot=off  SenseRDDot=off  SenseX=on  SenseY=on  SenseZ=on  SenseRad=on  SenseAzim=off  SenseDist=off  SenseInc=off  SenseXDot=off  SenseYDot=off  SenseZDot=off  SenseRadDot=off  SenseAzimDot=off  SenseDistDot=off  SenseIncDot=off  SenseXDDot=off  SenseYDDot=off  SenseZDDot=off  SenseRadDDot=off  SenseAzimDDot=off  SenseDistDDot=off  SenseIncDDot=off  BlockFunction=simmechanics.library.frames_transforms.transform_sensor
  base_coord_sys : PMIOPort  Port=1  Side=Left
  marker : PMIOPort  Port=2  Side=Left
  xyz : Outport
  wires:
  Mux/1 -> xyz/1
  Pos Y Converter/1 -> Mux/2
  Pos X Converter/1 -> Mux/1
  Pos Z Converter2/1 -> Mux/3
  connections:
  Transform Sensor/RConn3 -- Pos Y Converter/LConn1
  Pos X Converter/LConn1 -- Transform Sensor/RConn2
  Pos Z Converter2/LConn1 -- Transform Sensor/RConn4
  marker/RConn1 -- Transform Sensor/RConn1
  base_coord_sys/RConn1 -- Transform Sensor/LConn1

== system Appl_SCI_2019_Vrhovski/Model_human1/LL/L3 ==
  Mux : Mux  Inputs=3
  Pos X Converter : nesl_utility/PS-Simulink Converter  PhysicalDomain=network_engine_domain  SubClassName=ps_output  LeftPortType=input  RightPortType=output  PseudoPeriodic=off  Frequencies=[]  Unit=mm  AffineConversion=off
  Pos Y Converter : nesl_utility/PS-Simulink Converter  PhysicalDomain=network_engine_domain  SubClassName=ps_output  LeftPortType=input  RightPortType=output  PseudoPeriodic=off  Frequencies=[]  Unit=mm  AffineConversion=off
  Pos Z Converter2 : nesl_utility/PS-Simulink Converter  PhysicalDomain=network_engine_domain  SubClassName=ps_output  LeftPortType=input  RightPortType=output  PseudoPeriodic=off  Frequencies=[]  Unit=mm  AffineConversion=off
  Transform Sensor : sm_lib/Frames and Transforms/Transform Sensor  MeasurementFrame=World  SenseAngle=off  SenseAxis=off  SenseAngle1=off  SenseAngle2=off  SenseAngle3=off  SenseQ=off  SenseR=off  SenseOmegaX=off  SenseOmegaY=off  SenseOmegaZ=off  SenseOmega1=off  SenseOmega2=off  SenseOmega3=off  SenseQDot=off  SenseRDot=off  SenseAlphaX=off  SenseAlphaY=off  SenseAlphaZ=off  SenseAlpha1=off  SenseAlpha2=off  SenseAlpha3=off  SenseQDDot=off  SenseRDDot=off  SenseX=on  SenseY=on  SenseZ=on  SenseRad=on  SenseAzim=off  SenseDist=off  SenseInc=off  SenseXDot=off  SenseYDot=off  SenseZDot=off  SenseRadDot=off  SenseAzimDot=off  SenseDistDot=off  SenseIncDot=off  SenseXDDot=off  SenseYDDot=off  SenseZDDot=off  SenseRadDDot=off  SenseAzimDDot=off  SenseDistDDot=off  SenseIncDDot=off  BlockFunction=simmechanics.library.frames_transforms.transform_sensor
  base_coord_sys : PMIOPort  Port=1  Side=Left
  marker : PMIOPort  Port=2  Side=Left
  xyz : Outport
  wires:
  Pos Z Converter2/1 -> Mux/3
  Pos X Converter/1 -> Mux/1
  Pos Y Converter/1 -> Mux/2
  Mux/1 -> xyz/1
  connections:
  base_coord_sys/RConn1 -- Transform Sensor/LConn1
  marker/RConn1 -- Transform Sensor/RConn1
  Pos Z Converter2/LConn1 -- Transform Sensor/RConn4
  Pos X Converter/LConn1 -- Transform Sensor/RConn2
  Transform Sensor/RConn3 -- Pos Y Converter/LConn1

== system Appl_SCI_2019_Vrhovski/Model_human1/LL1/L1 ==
  Mux : Mux  Inputs=3
  Pos X Converter : nesl_utility/PS-Simulink Converter  PhysicalDomain=network_engine_domain  SubClassName=ps_output  LeftPortType=input  RightPortType=output  PseudoPeriodic=off  Frequencies=[]  Unit=mm  AffineConversion=off
  Pos Y Converter : nesl_utility/PS-Simulink Converter  PhysicalDomain=network_engine_domain  SubClassName=ps_output  LeftPortType=input  RightPortType=output  PseudoPeriodic=off  Frequencies=[]  Unit=mm  AffineConversion=off
  Pos Z Converter2 : nesl_utility/PS-Simulink Converter  PhysicalDomain=network_engine_domain  SubClassName=ps_output  LeftPortType=input  RightPortType=output  PseudoPeriodic=off  Frequencies=[]  Unit=mm  AffineConversion=off
  Transform Sensor : sm_lib/Frames and Transforms/Transform Sensor  MeasurementFrame=World  SenseAngle=off  SenseAxis=off  SenseAngle1=off  SenseAngle2=off  SenseAngle3=off  SenseQ=off  SenseR=off  SenseOmegaX=off  SenseOmegaY=off  SenseOmegaZ=off  SenseOmega1=off  SenseOmega2=off  SenseOmega3=off  SenseQDot=off  SenseRDot=off  SenseAlphaX=off  SenseAlphaY=off  SenseAlphaZ=off  SenseAlpha1=off  SenseAlpha2=off  SenseAlpha3=off  SenseQDDot=off  SenseRDDot=off  SenseX=on  SenseY=on  SenseZ=on  SenseRad=on  SenseAzim=off  SenseDist=off  SenseInc=off  SenseXDot=off  SenseYDot=off  SenseZDot=off  SenseRadDot=off  SenseAzimDot=off  SenseDistDot=off  SenseIncDot=off  SenseXDDot=off  SenseYDDot=off  SenseZDDot=off  SenseRadDDot=off  SenseAzimDDot=off  SenseDistDDot=off  SenseIncDDot=off  BlockFunction=simmechanics.library.frames_transforms.transform_sensor
  base_coord_sys : PMIOPort  Port=1  Side=Left
  marker : PMIOPort  Port=2  Side=Left
  xyz : Outport
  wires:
  Mux/1 -> xyz/1
  Pos Y Converter/1 -> Mux/2
  Pos X Converter/1 -> Mux/1
  Pos Z Converter2/1 -> Mux/3
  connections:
  Transform Sensor/RConn3 -- Pos Y Converter/LConn1
  Pos X Converter/LConn1 -- Transform Sensor/RConn2
  Pos Z Converter2/LConn1 -- Transform Sensor/RConn4
  marker/RConn1 -- Transform Sensor/RConn1
  base_coord_sys/RConn1 -- Transform Sensor/LConn1

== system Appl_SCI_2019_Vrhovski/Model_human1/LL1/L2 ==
  Mux : Mux  Inputs=3
  Pos X Converter : nesl_utility/PS-Simulink Converter  PhysicalDomain=network_engine_domain  SubClassName=ps_output  LeftPortType=input  RightPortType=output  PseudoPeriodic=off  Frequencies=[]  Unit=mm  AffineConversion=off
  Pos Y Converter : nesl_utility/PS-Simulink Converter  PhysicalDomain=network_engine_domain  SubClassName=ps_output  LeftPortType=input  RightPortType=output  PseudoPeriodic=off  Frequencies=[]  Unit=mm  AffineConversion=off
  Pos Z Converter2 : nesl_utility/PS-Simulink Converter  PhysicalDomain=network_engine_domain  SubClassName=ps_output  LeftPortType=input  RightPortType=output  PseudoPeriodic=off  Frequencies=[]  Unit=mm  AffineConversion=off
  Transform Sensor : sm_lib/Frames and Transforms/Transform Sensor  MeasurementFrame=World  SenseAngle=off  SenseAxis=off  SenseAngle1=off  SenseAngle2=off  SenseAngle3=off  SenseQ=off  SenseR=off  SenseOmegaX=off  SenseOmegaY=off  SenseOmegaZ=off  SenseOmega1=off  SenseOmega2=off  SenseOmega3=off  SenseQDot=off  SenseRDot=off  SenseAlphaX=off  SenseAlphaY=off  SenseAlphaZ=off  SenseAlpha1=off  SenseAlpha2=off  SenseAlpha3=off  SenseQDDot=off  SenseRDDot=off  SenseX=on  SenseY=on  SenseZ=on  SenseRad=on  SenseAzim=off  SenseDist=off  SenseInc=off  SenseXDot=off  SenseYDot=off  SenseZDot=off  SenseRadDot=off  SenseAzimDot=off  SenseDistDot=off  SenseIncDot=off  SenseXDDot=off  SenseYDDot=off  SenseZDDot=off  SenseRadDDot=off  SenseAzimDDot=off  SenseDistDDot=off  SenseIncDDot=off  BlockFunction=simmechanics.library.frames_transforms.transform_sensor
  base_coord_sys : PMIOPort  Port=1  Side=Left
  marker : PMIOPort  Port=2  Side=Left
  xyz : Outport
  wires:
  Pos Z Converter2/1 -> Mux/3
  Pos X Converter/1 -> Mux/1
  Pos Y Converter/1 -> Mux/2
  Mux/1 -> xyz/1
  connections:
  base_coord_sys/RConn1 -- Transform Sensor/LConn1
  marker/RConn1 -- Transform Sensor/RConn1
  Pos Z Converter2/LConn1 -- Transform Sensor/RConn4
  Pos X Converter/LConn1 -- Transform Sensor/RConn2
  Transform Sensor/RConn3 -- Pos Y Converter/LConn1

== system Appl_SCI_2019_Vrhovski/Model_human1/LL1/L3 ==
  Mux : Mux  Inputs=3
  Pos X Converter : nesl_utility/PS-Simulink Converter  PhysicalDomain=network_engine_domain  SubClassName=ps_output  LeftPortType=input  RightPortType=output  PseudoPeriodic=off  Frequencies=[]  Unit=mm  AffineConversion=off
  Pos Y Converter : nesl_utility/PS-Simulink Converter  PhysicalDomain=network_engine_domain  SubClassName=ps_output  LeftPortType=input  RightPortType=output  PseudoPeriodic=off  Frequencies=[]  Unit=mm  AffineConversion=off
  Pos Z Converter2 : nesl_utility/PS-Simulink Converter  PhysicalDomain=network_engine_domain  SubClassName=ps_output  LeftPortType=input  RightPortType=output  PseudoPeriodic=off  Frequencies=[]  Unit=mm  AffineConversion=off
  Transform Sensor : sm_lib/Frames and Transforms/Transform Sensor  MeasurementFrame=World  SenseAngle=off  SenseAxis=off  SenseAngle1=off  SenseAngle2=off  SenseAngle3=off  SenseQ=off  SenseR=off  SenseOmegaX=off  SenseOmegaY=off  SenseOmegaZ=off  SenseOmega1=off  SenseOmega2=off  SenseOmega3=off  SenseQDot=off  SenseRDot=off  SenseAlphaX=off  SenseAlphaY=off  SenseAlphaZ=off  SenseAlpha1=off  SenseAlpha2=off  SenseAlpha3=off  SenseQDDot=off  SenseRDDot=off  SenseX=on  SenseY=on  SenseZ=on  SenseRad=on  SenseAzim=off  SenseDist=off  SenseInc=off  SenseXDot=off  SenseYDot=off  SenseZDot=off  SenseRadDot=off  SenseAzimDot=off  SenseDistDot=off  SenseIncDot=off  SenseXDDot=off  SenseYDDot=off  SenseZDDot=off  SenseRadDDot=off  SenseAzimDDot=off  SenseDistDDot=off  SenseIncDDot=off  BlockFunction=simmechanics.library.frames_transforms.transform_sensor
  base_coord_sys : PMIOPort  Port=1  Side=Left
  marker : PMIOPort  Port=2  Side=Left
  xyz : Outport
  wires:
  Mux/1 -> xyz/1
  Pos Y Converter/1 -> Mux/2
  Pos X Converter/1 -> Mux/1
  Pos Z Converter2/1 -> Mux/3
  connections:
  Transform Sensor/RConn3 -- Pos Y Converter/LConn1
  Pos X Converter/LConn1 -- Transform Sensor/RConn2
  Pos Z Converter2/LConn1 -- Transform Sensor/RConn4
  marker/RConn1 -- Transform Sensor/RConn1
  base_coord_sys/RConn1 -- Transform Sensor/LConn1
